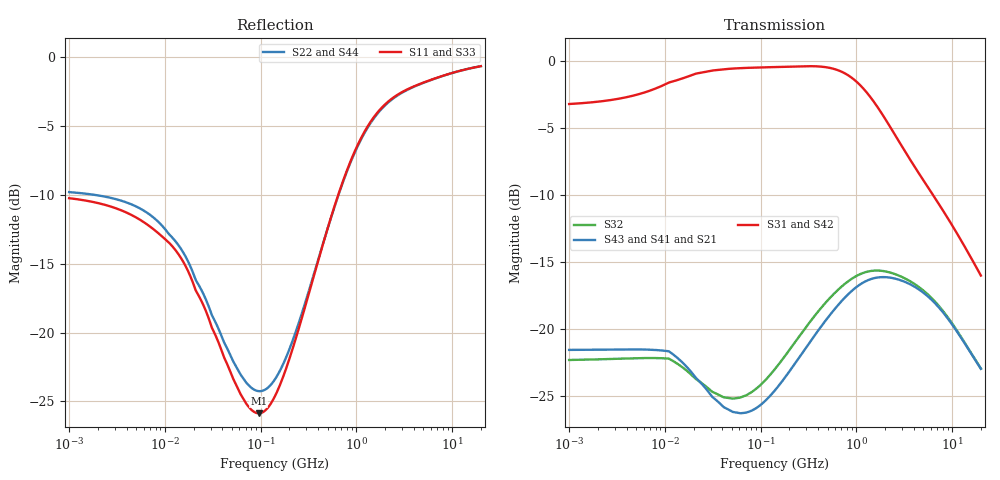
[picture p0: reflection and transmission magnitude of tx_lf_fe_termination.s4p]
! Created Wed Jul 29 12:30:48 2015
# hz S db R 50
! 4 Port Network Data from SP1.SP block
! freq  dbS11  angS11  dbS12  angS12  dbS13  angS13  dbS14  angS14
!  dbS21  angS21  dbS22  angS22  dbS23  angS23  dbS24  angS24
!  dbS31  angS31  dbS32  angS32  dbS33  angS33  dbS34  angS34
!  dbS41  angS41  dbS42  angS42  dbS43  angS43  dbS44  angS44
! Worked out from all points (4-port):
!   861 points, 1 MHz to 20 GHz, reference 50 ohm
!   strongest paths, dB at 1 MHz, 11.89 MHz, 141.4 MHz, 1.682 GHz, 20 GHz:
!     S31: -3.2, -1.5, -0.4, -3.5, -16.0
!     S42: -3.4, -1.7, -0.5, -3.5, -16.0
!     S43: -21.6, -21.8, -24.6, -16.1, -23.0
!     S41: -21.6, -21.8, -24.6, -16.1, -23.0
!     S21: -21.6, -21.8, -24.6, -16.1, -23.0
!     S32: -22.3, -22.3, -23.0, -15.6, -22.9
!   lowest |S11| = -25.9 dB at 95.6 MHz (marker M1), VSWR 1.11, Z = 45.2 - j0.622 ohm
!   |S11| at or under -10 dB: start of sweep to 646.3 MHz
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1000000  -10.23 175.2  -22.31 -3.3  -3.18 2.1  -22.31 -3.3
         -21.55 -2.7  -9.79 175.5  -21.55 -2.7  -3.38 2.2
         -3.18 2.1  -22.31 -3.3  -10.23 175.2  -22.31 -3.3
         -21.55 -2.7  -3.38 2.2  -21.55 -2.7  -9.79 175.5
1.189207e7  -13.70 144.4  -22.34 -52.9  -1.51 8.2  -22.34 -52.9
            -21.83 -47.3  -13.07 146.1  -21.83 -47.3  -1.67 8.6
            -1.51 8.2  -22.34 -52.9  -13.70 144.4  -22.34 -52.9
            -21.83 -47.3  -1.67 8.6  -21.83 -47.3  -13.07 146.1
9.560361e7  -25.87 -172.3  -24.29 -138.1  -0.45 -0.4  -24.29 -138.1
            -25.77 -132.5  -24.25 -174.5  -25.77 -132.5  -0.55 -0.4
            -0.45 -0.4  -24.29 -138.1  -25.87 -172.3  -24.29 -138.1
            -25.77 -132.5  -0.55 -0.4  -25.77 -132.5  -24.25 -174.5
5.077477e8  -12.30 -109.0  -17.81 151.6  -0.45 -14.0  -17.81 151.6
            -19.11 148.7  -12.31 -112.3  -19.11 148.7  -0.58 -13.9
            -0.45 -14.0  -17.81 151.6  -12.30 -109.0  -17.81 151.6
            -19.11 148.7  -0.58 -13.9  -19.11 148.7  -12.31 -112.3
1.366945e9  -4.82 -132.4  -15.67 73.4  -2.56 -34.7  -15.67 73.4
            -16.30 69.7  -4.91 -133.3  -16.30 69.7  -2.65 -34.1
            -2.56 -34.7  -15.67 73.4  -4.82 -132.4  -15.67 73.4
            -16.30 69.7  -2.65 -34.1  -16.30 69.7  -4.91 -133.3
3.722675e9  -2.20 -156.3  -16.46 9.7  -7.43 -47.2  -16.46 9.7
            -16.68 8.4  -2.23 -156.4  -16.68 8.4  -7.43 -46.8
            -7.43 -47.2  -16.46 9.7  -2.20 -156.3  -16.46 9.7
            -16.68 8.4  -7.43 -46.8  -16.68 8.4  -2.23 -156.4
2e10  -0.63 -171.6  -22.95 -42.5  -16.00 -59.5  -22.95 -42.5
      -22.97 -42.4  -0.63 -171.5  -22.97 -42.4  -15.99 -59.5
      -16.00 -59.5  -22.95 -42.5  -0.63 -171.6  -22.95 -42.5
      -22.97 -42.4  -15.99 -59.5  -22.97 -42.4  -0.63 -171.5
